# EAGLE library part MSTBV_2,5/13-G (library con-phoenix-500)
Grundleiste - MSTBV 2,5/13-G - 1753657 Grundgehäuse, Nennstrom: 12 A Bemessungsspannung (III/2): 320 V Polzahl: 13 Rastermaß: 5 mm Farbe: grün Kontaktoberfläche: Zinn Montage: Löten
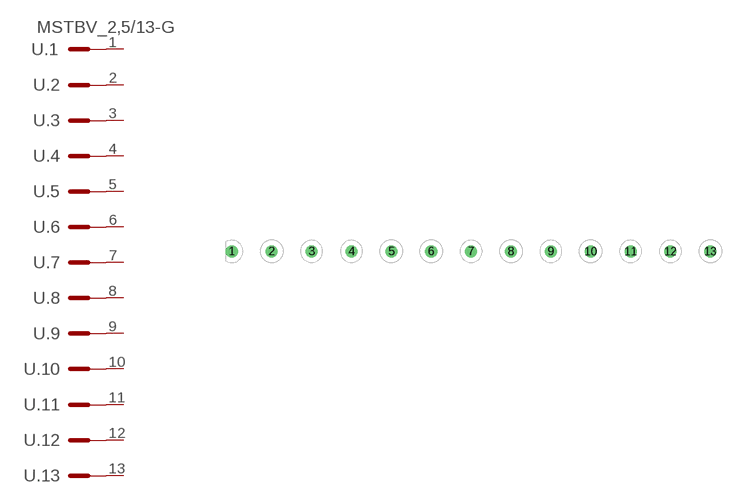
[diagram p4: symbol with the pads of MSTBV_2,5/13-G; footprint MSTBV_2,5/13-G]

Designator prefix -; gates .1=PIN+V .2=PIN .3=PIN .4=PIN .5=PIN .6=PIN .7=PIN .8=PIN .9=PIN .10=PIN .11=PIN .12=PIN .13=PIN

## MSTBV_2,5/13-G  [MSTBV_2,5/13-G]
1  .1:SK  pas
2  .2:SK  pas
3  .3:SK  pas
4  .4:SK  pas
5  .5:SK  pas
6  .6:SK  pas
7  .7:SK  pas
8  .8:SK  pas
9  .9:SK  pas
10  .10:SK  pas
11  .11:SK  pas
12  .12:SK  pas
13  .13:SK  pas

## Footprint MSTBV_2,5/13-G (pad centres in mm)
Grundleiste - MSTBV 2,5/13-G - 1753657 Grundgehäuse, Nennstrom: 12 A Bemessungsspannung (III/2): 320 V Polzahl: 13 Rastermaß: 5 mm Farbe: grün Kontaktoberfläche: Zinn Montage: Löten
drill 1 pad 1.422: 1 -30,0; 2 -25,0; 3 -20,0; 4 -15,0; 5 -10,0; 6 -5,0; 7 0,0; 8 5,0; 9 10,0; 10 15,0; 11 20,0; 12 25,0; 13 30,0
